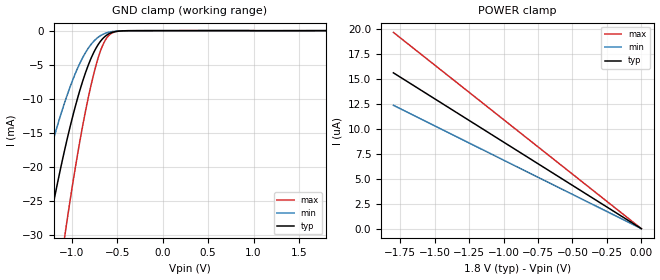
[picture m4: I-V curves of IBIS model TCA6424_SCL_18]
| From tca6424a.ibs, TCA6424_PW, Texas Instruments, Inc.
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[Model]   TCA6424_SCL_18
Model_type  Input
Vinl=0.495
Vinh=1.365
| variable   typ   min   max
C_comp   2.17pF   1.62pF   2.41pF
[Temperature Range]   40   100   -40
| Ambient temperature   25   85   -40
[Voltage range]   1.8   1.65   1.95
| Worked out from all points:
|   GND clamp passes 1 mA (typ) near -0.65 V on its own axis
[GND Clamp]
| TCA6424_SCL_18
|   Voltage   I(typ)   I(min)   I(max)
-1.8V     -74.03mA   -51.67mA   -111.7mA
-1.45V    -43.77mA   -29.21mA   -69.33mA
-1.27V    -30.12mA   -19.36mA   -49.42mA
-1.25V    -28.71mA   -18.36mA   -47.32mA
-1.07V    -17.07mA   -10.25mA   -29.6mA
-960mV    -11.11mA   -6.286mA   -20.1mA
-855mV    -6.443mA   -3.38mA    -12.28mA
-765mV    -3.411mA   -1.671mA   -6.762mA
-680mV    -1.503mA   -712.5uA   -2.841mA
-590mV    -455.1uA   -232.6uA   -683.2uA
-475mV    -59.06uA   -41.09uA   -61.18uA
1.8V      147.6pA    1.03uA     -1.64uA
[POWER Clamp]
| TCA6424_SCL_18
|   Voltage   I(typ)   I(min)   I(max)
-1.8V     15.63uA    12.37uA    19.68uA
-1.5V     13.02uA    10.31uA    16.4uA
-830mV    7.204uA    5.702uA    9.075uA
-16.28fV  147.6pA    508.2pA    35.05pA
